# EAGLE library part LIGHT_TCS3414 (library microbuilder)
Taos TCS3414CS Digital Colour Light Sensor Mouser: 856-TCS3414CS
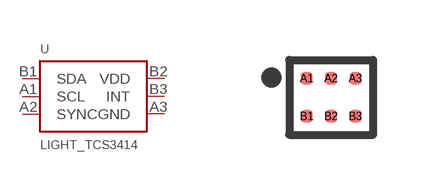
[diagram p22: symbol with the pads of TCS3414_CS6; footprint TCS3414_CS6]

Designator prefix U

## LIGHT_TCS3414  [TCS3414_CS6]
A1  SCL
A2  SYNC
A3  GND
B1  SDA
B2  VDD
B3  INT

## Footprint TCS3414_CS6 (pad centres in mm)
6 Lead Chipscale 0.30mm pads, 0.61mm pitch Source: http://www.taosinc.com/getfile.aspx?type=press&file=tcs3404cs-e46.pdf
smd 0.3 x 0.3: A1 -0.61,0.475; A2 0,0.475; A3 0.61,0.475; B1 -0.61,-0.475; B2 0,-0.475; B3 0.61,-0.475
